DATA_BLOCK DB 1
TITLE =
VERSION : 0.1


  STRUCT
   aa { S7_m_c := 'true' }: BOOL ;	//aa
   aa1 { S7_m_c := 'true' }: BYTE  := B#16#1;	//bb
   aa2 { S7_m_c := 'true' }: WORD  := W#16#2;	//cc
   aa3 { S7_m_c := 'true' }: DWORD  := DW#16#3;	//dd
   aa4 { S7_m_c := 'true' }: REAL  := 4.000000e+000;	//ee
   aa5 { S7_m_c := 'true' }: INT  := 5;	//ff
   aa6 { S7_m_c := 'true' }: DINT  := L#6;	//gg
   aa7 { S7_m_c := 'true' }: INT  := 7;	//hh
   aa8 { S7_m_c := 'true' }: INT  := 8;	//Temporary placeholder variable
   aa9 { S7_m_c := 'true' }: INT  := 9;	//Temporary placeholder variable
   aa10 { S7_m_c := 'true' }: INT  := 10;	//Temporary placeholder variable
  END_STRUCT ;
BEGIN
   aa := FALSE;
   aa1 := B#16#1;
   aa2 := W#16#2;
   aa3 := DW#16#3;
   aa4 := 4.000000e+000;
   aa5 := 66;
   aa6 := L#6;
   aa7 := 88;
   aa8 := 99;
   aa9 := 100;
   aa10 := 1000;
END_DATA_BLOCK

